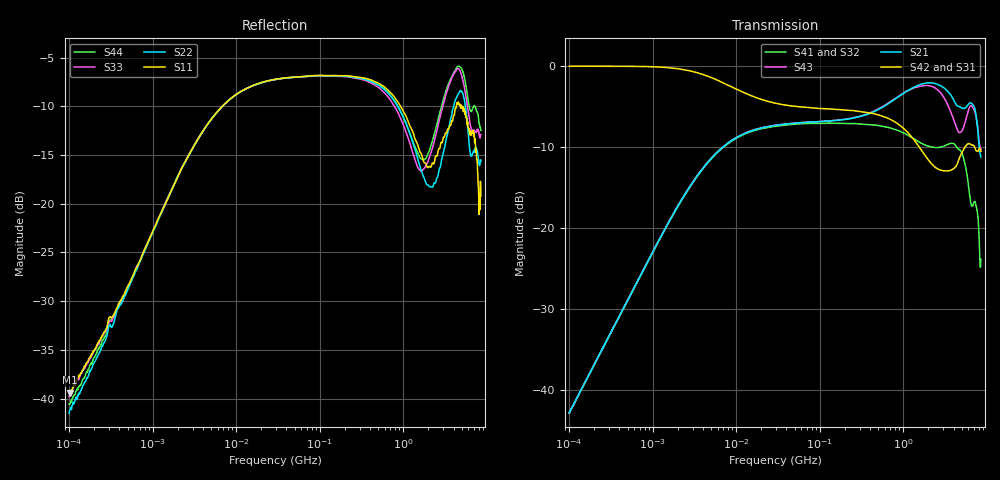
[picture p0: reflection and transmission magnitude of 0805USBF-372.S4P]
# Hz S dB R 50
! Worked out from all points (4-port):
!   801 points, 100 kHz to 8.5 GHz, reference 50 ohm
!   strongest paths, dB at 100 kHz, 1.721 MHz, 29.51 MHz, 502.3 MHz, 8.5 GHz:
!     S42: 0.0, -0.3, -4.6, -6.0, -10.5
!     S31: -0.1, -0.3, -4.6, -6.1, -10.6
!     S21: -42.9, -18.5, -7.3, -5.4, -11.3
!     S43: -42.9, -18.5, -7.3, -5.3, -10.3
!     S41: -42.9, -18.6, -7.5, -7.4, -23.9
!     S32: -43.0, -18.6, -7.5, -7.5, -26.6
!   lowest |S11| = -39.4 dB at 101.7 kHz (marker M1), VSWR 1.02, Z = 50.3 + j1.03 ohm
!   |S11| at or under -10 dB: 929 MHz to 4.322 GHz (3.393 GHz wide, 129 % of centre); 4.969 GHz to 5.161 GHz (191.7 MHz wide, 3.79 % of centre); 5.162 GHz to end of sweep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
100000  -39.29 72.7  -42.85 88.2  -0.06 -0.5  -42.88 -91.6
        -42.86 88.3  -41.51 66.1  -43.04 -91.7  -0.03 -0.4
        -0.05 -0.5  -42.96 -91.2  -39.80 59.2  -42.84 88.2
        -42.92 -92.0  -0.03 -0.4  -42.93 88.7  -40.59 71.3
101665  -39.40 72.6  -42.67 88.5  -0.06 -0.5  -42.79 -91.8
        -42.69 88.2  -41.21 66.1  -42.86 -91.8  -0.03 -0.4
        -0.05 -0.5  -42.84 -91.9  -39.61 58.8  -42.73 88.4
        -42.84 -91.8  -0.03 -0.4  -42.81 88.2  -40.61 72.9
1.471637e7  -7.98 21.3  -8.07 22.3  -3.67 -17.4  -8.13 -159.6
            -8.09 22.3  -8.00 21.2  -8.20 -159.5  -3.66 -17.6
            -3.66 -17.4  -8.20 -159.4  -7.99 21.0  -8.05 22.1
            -8.15 -159.4  -3.63 -17.6  -8.04 22.2  -7.99 21.4
1.187242e9  -11.90 141.6  -2.91 177.6  -8.46 103.0  -8.67 -83.1
            -2.92 177.6  -12.72 136.8  -8.78 -87.2  -8.44 103.2
            -8.46 102.9  -8.78 -87.2  -13.65 146.1  -2.95 175.0
            -8.67 -83.0  -8.45 103.2  -2.95 175.0  -12.67 148.0
2.16292e9  -16.18 1.2  -2.08 4.0  -11.94 -93.8  -10.01 83.1
           -2.09 3.9  -18.27 7.0  -10.19 77.5  -12.05 -89.9
           -11.92 -93.8  -10.18 77.5  -14.71 27.4  -2.50 -0.4
           -10.00 83.1  -12.06 -90.1  -2.50 -0.4  -13.95 24.7
3.154505e9  -12.97 -137.5  -2.80 -169.6  -12.97 60.0  -9.85 -107.8
            -2.81 -169.7  -14.07 -129.9  -9.81 -115.3  -12.96 67.0
            -12.96 59.9  -9.81 -115.3  -9.16 -133.0  -4.12 -175.7
            -9.83 -107.7  -12.96 66.9  -4.12 -175.7  -8.78 -126.4
8.5e9  -19.21 55.1  -11.26 21.2  -10.62 75.1  -24.67 -69.5
       -11.27 21.2  -15.65 -4.7  -26.67 -109.3  -10.56 75.4
       -10.58 75.0  -26.62 -109.4  -12.91 -37.3  -10.27 32.5
       -23.91 -71.9  -10.55 75.0  -10.26 32.6  -12.47 -7.8
